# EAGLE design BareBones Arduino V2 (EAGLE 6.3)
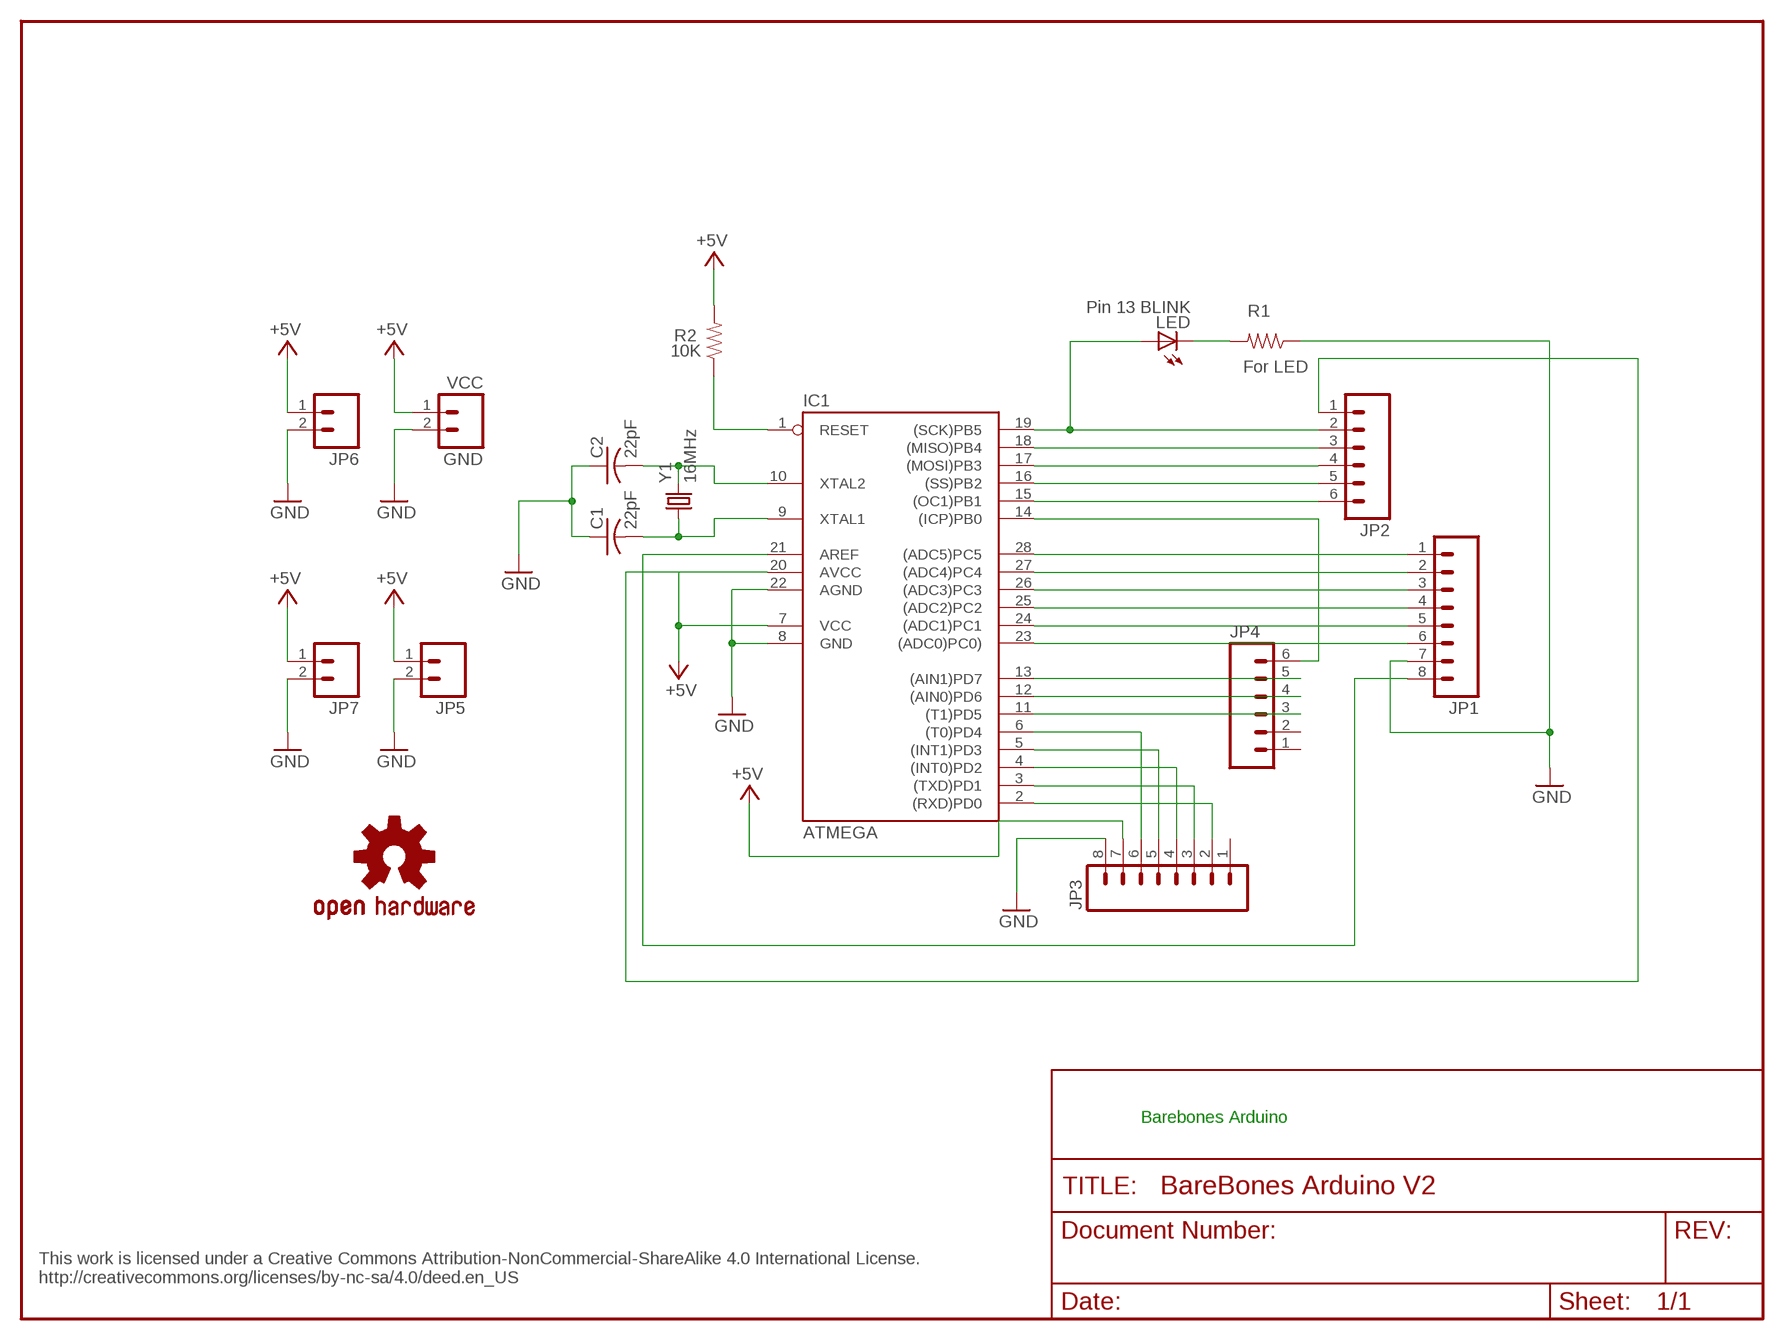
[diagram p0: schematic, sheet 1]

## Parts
C1  22pF  C-US025-024X044  [C025-024X044]
C2  22pF  C-US025-024X044  [C025-024X044]
GND  VCC  M02PTH  [1X02]
IC1  ATMEGA  AT90S4433P  [DIL28-3]
JP1  M081X08  [1X08]
JP2  M06SIP  [1X06]
JP3  M081X08  [1X08]
JP4  M06SIP  [1X06]
JP5  M02PTH  [1X02]
JP6  M02PTH  [1X02]
JP7  M02PTH  [1X02]
LED  Pin 13 BLINK  LED3MM  [LED3MM]
R1  For LED  RESISTORPTH-1/4W  [AXIAL-0.4]
R2  10K  RESISTORPTH-1/4W  [AXIAL-0.4]
U$1  OSHW-LOGOS  [OSHW-LOGO-S]
Y1  16MHz  CRYSTALHC49US  [HC49US]

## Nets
+5V [power]: GND.1 IC1.7(VCC) IC1.20(AVCC) JP2.1 JP3.7 JP5.1 JP6.1 JP7.1 R2.P$2
GND [power]: C1.1 C2.1 GND.2 IC1.8(GND) IC1.22(AGND) JP1.7 JP3.8 JP5.2 JP6.2 JP7.2 R1.P$1
M8RXD: IC1.2((RXD)PD0) JP3.2
N$1: IC1.18((MISO)PB4) JP2.3
N$2: IC1.1(RESET) R2.P$1
N$3: IC1.24((ADC1)PC1) JP1.5
N$4: IC1.17((MOSI)PB3) JP2.4
N$5: IC1.11((T1)PD5) JP4.3
N$6: C1.2 IC1.9(XTAL1) Y1.1
N$7: C2.2 IC1.10(XTAL2) Y1.2
N$8: LED.K(C) R1.P$2
N$9: IC1.3((TXD)PD1) JP3.3
N$10: IC1.4((INT0)PD2) JP3.4
N$11: IC1.5((INT1)PD3) JP3.5
N$12: IC1.6((T0)PD4) JP3.6
N$13: IC1.12((AIN0)PD6) JP4.4
N$14: IC1.13((AIN1)PD7) JP4.5
N$15: IC1.14((ICP)PB0) JP4.6
N$16: IC1.15((OC1)PB1) JP2.6
N$17: IC1.16((SS)PB2) JP2.5
N$18: IC1.23((ADC0)PC0)) JP1.6
N$19: IC1.25((ADC2)PC2) JP1.4
N$20: IC1.26((ADC3)PC3) JP1.3
N$21: IC1.27((ADC4)PC4) JP1.2
N$22: IC1.28((ADC5)PC5) JP1.1
N$23: IC1.21(AREF) JP1.8
SCK: IC1.19((SCK)PB5) JP2.2 LED.A
Unconnected: JP3.1 JP4.1 JP4.2

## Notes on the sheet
- Barebones Arduino
- This work is licensed under a Creative Commons Attribution-NonCommercial-ShareAlike 4.0 International License.
  http://creativecommons.org/licenses/by-nc-sa/4.0/deed.en_US

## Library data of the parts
C1 C2 = adafruit:C-US: CAPACITOR, American symbol
GND JP5-JP7 = SparkFun:M02: Header 2
IC1 = atmel:AT90S4433: MICROCONTROLLER 4 Kbytes FLASH 128 bytes SRAM 256 bytes EEPROM UART 6-channel 10 bit ADC
JP1 JP3 = SparkFun:M08: Header 8 Standard 8-pin 0.1" header. Use with straight break away headers (SKU : PRT-00116), right angle break away headers (PRT-00553), swiss pins (PRT-00743), machine pins (PRT-00117), and female headers (PRT-00115).
JP2 JP4 = SparkFun:M06: Header 6 Standard 6-pin 0.1" header. Use with straight break away headers (SKU : PRT-00116), right angle break away headers (PRT-00553), swiss pins (PRT-00743), machine pins (PRT-00117), and female headers (PRT-00115). Molex polarized connector foot print use with SKU : PRT-08094 with associated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
LED = adafruit:LED: LED
R1 R2 = SparkFun:RESISTOR: Resistor
U$1 = SparkFun:OSHW-LOGO: Open Source Hardware Logo This logo indicates the piece of hardware it is found on incorporates a OSHW license and/or adheres to the definition of open source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
Y1 = SparkFun:CRYSTAL: Crystals

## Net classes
0 default: width 0.4 mm, clearance 0.3 mm
1 power: width 0.6 mm, clearance 0.3 mm

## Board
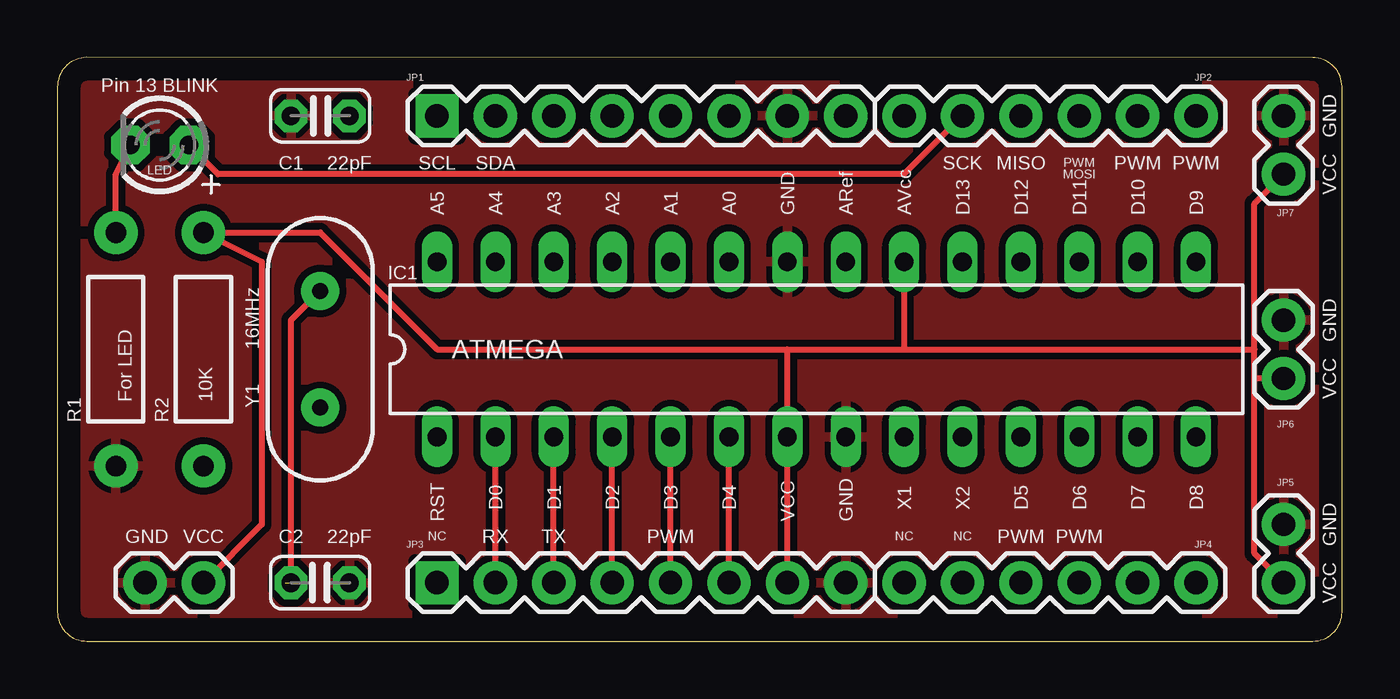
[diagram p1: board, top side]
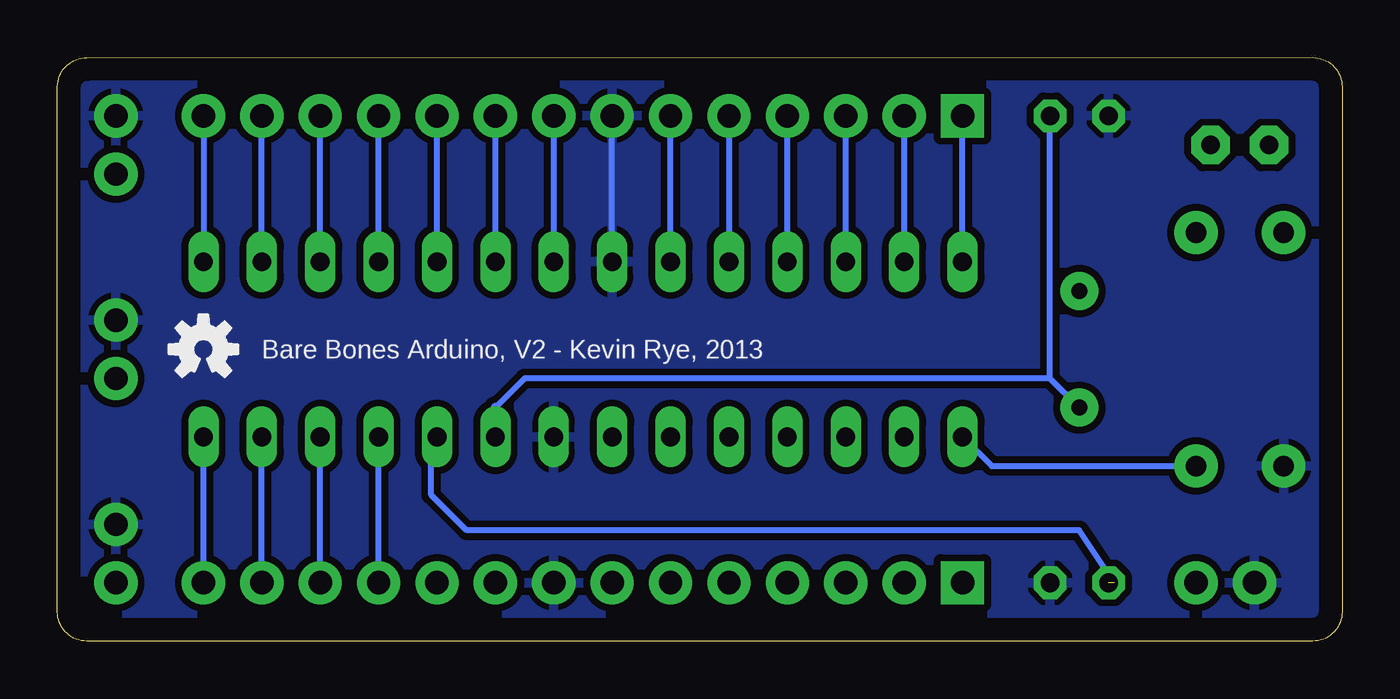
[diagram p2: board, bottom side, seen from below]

Size 55.88 x 25.4 mm. Coordinates in mm from the lower left corner, seen from the top.
Outline: 0,24.12 0,1.27 arc90 1.27,0 54.61,0 arc90 55.88,1.27 55.88,24.13 arc90 54.61,25.39 1.27,25.4 arc90 0,24.12
Copper layers (1*16): Top 0.035mm / dielectric 1.5mm / Bottom 0.035mm
Design rules "default": minimum track width 10mil, minimum drill 24mil, track to track 8mil, track to pad 8mil, pad to pad 8mil, via to via 8mil, smd to smd 8mil, copper to edge 40mil, drill to drill 8mil, minimum pad ring 10mil, minimum via ring 8mil, stop-mask expansion 4mil, vias tented up to drill 0mil, thermal gap 10mil

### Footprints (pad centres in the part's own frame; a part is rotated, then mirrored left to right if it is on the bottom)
C025-024X044 = drill 0.813 pad 1.422 octagon: 1 -1.27,0; 2 1.27,0
1X02 = drill 1.016 pad 1.88: 1 0,0; 2 2.54,0
DIL28-3 = drill 0.813 long: 1 -16.51,-3.81; 2 -13.97,-3.81; 3 -11.43,-3.81; 4 -8.89,-3.81; 5 -6.35,-3.81; 6 -3.81,-3.81; 7 -1.27,-3.81; 8 1.27,-3.81; 9 3.81,-3.81; 10 6.35,-3.81; 11 8.89,-3.81; 12 11.43,-3.81; 13 13.97,-3.81; 14 16.51,-3.81; 15 16.51,3.81; 16 13.97,3.81; 17 11.43,3.81; 18 8.89,3.81; 19 6.35,3.81; 20 3.81,3.81; 21 1.27,3.81; 22 -1.27,3.81; 23 -3.81,3.81; 24 -6.35,3.81; 25 -8.89,3.81; 26 -11.43,3.81; 27 -13.97,3.81; 28 -16.51,3.81
1X08 = drill 1.016 pad 1.88 square: 1 0,0 | drill 1.016 pad 1.88: 2 2.54,0; 3 5.08,0; 4 7.62,0; 5 10.16,0; 6 12.7,0; 7 15.24,0; 8 17.78,0
1X06 = drill 1.016 pad 1.88: 1 0,0; 2 2.54,0; 3 5.08,0; 4 7.62,0; 5 10.16,0; 6 12.7,0
LED3MM = drill 0.813 pad 1.676 octagon: A -1.27,0; K 1.27,0
AXIAL-0.4 = drill 0.9 pad 1.88: P$1 -5.08,0; P$2 5.08,0
HC49US = drill 0.7 pad 1.651: 1 -2.54,0; 2 2.54,0

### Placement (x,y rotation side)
C1  11.43,22.86 0 top
C2  11.43,2.54 180 top
GND  6.35,2.54 180 top
IC1  33.02,12.7 0 top
JP1  16.51,22.86 0 top
JP2  36.83,22.86 0 top
JP3  16.51,2.54 0 top
JP4  36.83,2.54 0 top
JP5  53.34,2.54 90 top
JP6  53.34,11.43 90 top
JP7  53.34,20.32 90 top
LED  4.44,21.59 180 top
R1  2.54,12.7 90 top
R2  6.35,12.7 90 top
U$1  49.53,12.7 0 bottom
Y1  11.43,12.7 90 top

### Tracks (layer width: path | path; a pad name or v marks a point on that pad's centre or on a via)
+5V
  Top 0.254: JP5.1 52.07,3.81 52.07,11.43 | 52.07,11.43 52.07,12.7 | 52.07,12.7 52.07,19.05 JP7.1 | IC1.20 36.83,12.7 | 36.83,12.7 52.07,12.7 | 31.75,12.7 IC1.7 JP3.7 | 31.75,12.7 36.83,12.7 | 31.75,12.7 16.51,12.7 11.43,17.78 R2.P$2 8.89,16.51 8.89,5.08 GND.1 | JP6.1 52.07,11.43
  Bottom 0.254: IC1.20 JP2.1
GND
  Bottom 0.254: IC1.22 JP1.7
  pour Top: -2.54,27.94 58.42,27.94 58.42,-2.54 -2.54,-2.54
  pour Bottom: -2.54,27.94 58.42,27.94 58.42,-2.54 -2.54,-2.54
M8RXD
  Top 0.254: JP3.2 IC1.2
N$1
  Bottom 0.254: IC1.18 JP2.3
N$2
  Bottom 0.254: IC1.1 15.24,7.62 R2.P$1
N$3
  Bottom 0.254: JP1.5 IC1.24
N$4
  Bottom 0.254: IC1.17 JP2.4
N$5
  Bottom 0.254: JP4.3 IC1.11
N$6
  Bottom 0.254: 12.7,11.43 12.7,22.73 C1.2 | Y1.1 12.7,11.43 | 12.7,11.43 35.56,11.43 36.83,10.16
  Bottom 0.406: 36.83,10.16 IC1.9
N$7  (1 unrouted)
  Top 0.254: C2.2 10.16,2.67 10.16,13.97 Y1.2
  Bottom 0.254: IC1.10 39.62,8.64 39.62,6.37 38.08,4.83 11.43,4.83 9.91,2.54
N$8
  Top 0.254: R1.P$2 2.54,20.32 LED.K
N$9
  Top 0.254: JP3.3 IC1.3
N$10
  Top 0.254: JP3.4 IC1.4
N$11
  Top 0.254: JP3.5 IC1.5
N$12
  Top 0.254: JP3.6 IC1.6
N$13
  Bottom 0.254: JP4.4 IC1.12
N$14
  Bottom 0.254: JP4.5 IC1.13
N$15
  Bottom 0.254: JP4.6 IC1.14
N$16
  Bottom 0.254: JP2.6 IC1.15
N$17
  Bottom 0.254: IC1.16 JP2.5
N$18
  Bottom 0.254: IC1.23 JP1.6
N$19
  Bottom 0.254: IC1.25 JP1.4
N$20
  Bottom 0.254: IC1.26 JP1.3
N$21
  Bottom 0.254: JP1.2 IC1.27
N$22
  Bottom 0.254: IC1.28 JP1.1
N$23
  Bottom 0.254: JP1.8 IC1.21
SCK
  Top 0.254: JP2.2 36.83,20.32 6.99,20.32 LED.A
  Bottom 0.254: IC1.19 JP2.2

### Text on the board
Unrouted: This work is licensed under a Creative Commons Attribution-NonCommercial-ShareAlike 4.0 International License. / http://creativecommons.org/licenses/by-nc-sa/4.0/deed.en_US
tNames: GND | C1 | 22pF | SCL | SDA | SCK | MISO | MOSI | PWM | PWM | PWM | VCC | A5 | A4 | A3 | A2 | A1 | A0 | GND | ARef | AVcc | D13 | D12 | D11 | D10 | D9 | GND | VCC | D0 | D1 | D2 | D3 | D4 | X1 | X2 | D5 | D6 | D7 | D8 | C2 | 22pF | NC | RST | RX | TX | PWM | VCC | GND | NC | NC | PWM | PWM | GND | VCC
bNames: Bare Bones Arduino, V2 - Kevin Rye, 2013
